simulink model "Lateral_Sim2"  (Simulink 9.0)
settings: Solver=ode45  StartTime=0.0  StopTime=80  RelTol=1e-3  EnableMultiTasking=on
InitFcn:
  | init_lat;
StopFcn:
  | pl
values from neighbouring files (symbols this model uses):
  Cyb = -0.023    [init_lat.m]    (also in init.m; init_pitch.m)
  Cyda = 0.0011    [init_lat.m]    (also in init.m; init_pitch.m)
  Cydr = 0.0034    [init_lat.m]    (also in init.m; init_pitch.m)
  d2r = pi/180    (= 0.0174532925199)    [frequ.m]    (also in init_lat.m; pl.m; init.m; freq.m)
  Mv = 1219.1    [init_lat.m]    (also in init.m; init_pitch.m)
  Qbar = 1220.6    [init_lat.m]    (also in init.m; init_pitch.m)
  Sref = 145.4    [init_lat.m]    (also in init.m; init_pitch.m)
undefined symbols (not defined in the file or in its folder): Al, Bl, Cl, Dl, Kpr

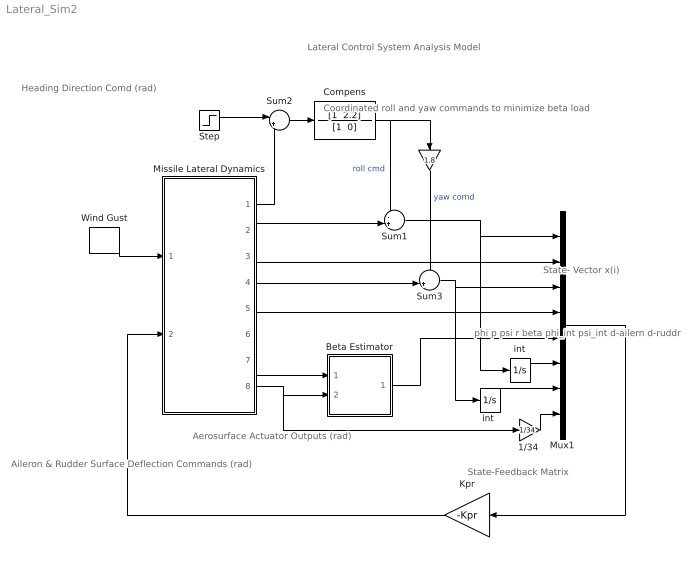
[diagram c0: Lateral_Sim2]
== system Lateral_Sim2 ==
  note: phi p psi r beta phi_int psi_int d-ailern d-ruddr
  note: Heading Direction Comd (rad)
  note: State- Vector x(i)
  note: Aileron & Rudder Surface Deflection Commands (rad)
  note: Aerosurface Actuator Outputs (rad)
  note: Coordinated roll and yaw commands to minimize beta load
  note: State-Feedback Matrix
  note: Lateral Control System Analysis Model
  " " : Gain  Gain=1.8
  "1/34 " : Gain  Gain=1/34
  Beta Estimator : Subsystem
  Compens : TransferFcn  Numerator="[1  2.2]"  Denominator="[1  0]"
  Kpr : Gain  Gain=-Kpr  Multiplication=Matrix(K*u)
  Missile Lateral Dynamics : Subsystem
  Mux1 : Mux  Inputs=[1, 1, 1, 1, 1, 1, 1, 2]
  Step : Step  Time=0  After=10*d2r  SampleTime=0
  Sum1 : Sum  Inputs=-+|
  Sum2 : Sum  Inputs=|+-
  Sum3 : Sum  Inputs=-+|
  Wind Gust : DiscretePulseGenerator  PulseType=Time based  Amplitude=30  Period=100  PulseWidth=5  PhaseDelay=10
  int : Integrator
  "int " : Integrator
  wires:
  Missile Lateral Dynamics/3(p) -> Mux1/2
  Missile Lateral Dynamics/5(r) -> Mux1/4
  Kpr/1 -> Missile Lateral Dynamics/2(aero)
  Sum1/1 -> Mux1/1, int/1
  Missile Lateral Dynamics/2(phi) -> Sum1/2
  Sum2/1 -> Compens/1
  int/1 -> Mux1/6
  Missile Lateral Dynamics/1(" Head") -> Sum2/2
  Compens/1 -> Sum1/1, " "/1  "roll cmd"
  Missile Lateral Dynamics/4(psi) -> Sum3/2
  Sum3/1 -> Mux1/3, "int "/1
  "int "/1 -> Mux1/7
  " "/1 -> Sum3/1  "yaw comd"
  Missile Lateral Dynamics/8(aeros) -> "1/34 "/1, Beta Estimator/2(delta)
  Mux1/1 -> Kpr/1
  "1/34 "/1 -> Mux1/8
  Missile Lateral Dynamics/7(Ny) -> Beta Estimator/1(Ny)
  Beta Estimator/1(beta) -> Mux1/5
  Wind Gust/1 -> Missile Lateral Dynamics/1(Gust)
  Step/1 -> Sum2/1

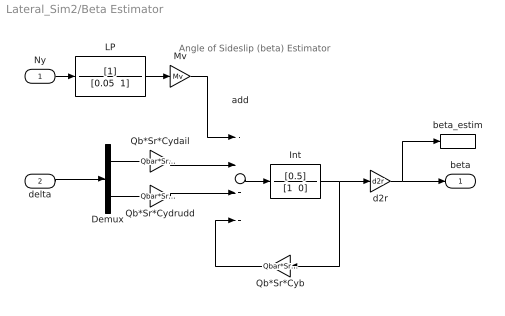
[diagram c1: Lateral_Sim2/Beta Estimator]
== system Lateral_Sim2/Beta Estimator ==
  note: Angle of Sideslip (beta) Estimator
  Ny : Inport
  delta : Inport  Port=2
  Demux : Demux  Outputs=2
  Int : TransferFcn  Numerator=[0.5]  Denominator="[1  0]"
  LP : TransferFcn  Denominator="[0.05  1]"
  Mv : Gain  Gain=Mv
  Qb*Sr*Cyb : Gain  Gain=Qbar*Sref*Cyb*1.2
  Qb*Sr*Cydail : Gain  Gain=Qbar*Sref*Cyda
  Qb*Sr*Cydrudd : Gain  Gain=Qbar*Sref*Cydr
  add : Sum  Inputs=-+++
  beta_estim : ToWorkspace  VariableName=betest  SampleTime=-1
  d2r : Gain  Gain=d2r
  beta : Outport
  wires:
  LP/1 -> Mv/1
  Qb*Sr*Cydail/1 -> add/2
  Qb*Sr*Cydrudd/1 -> add/3
  Qb*Sr*Cyb/1 -> add/4
  Ny/1 -> LP/1
  Int/1 -> d2r/1, Qb*Sr*Cyb/1
  d2r/1 -> beta_estim/1, beta/1
  Mv/1 -> add/1
  add/1 -> Int/1
  Demux/1 -> Qb*Sr*Cydail/1
  Demux/2 -> Qb*Sr*Cydrudd/1
  delta/1 -> Demux/1

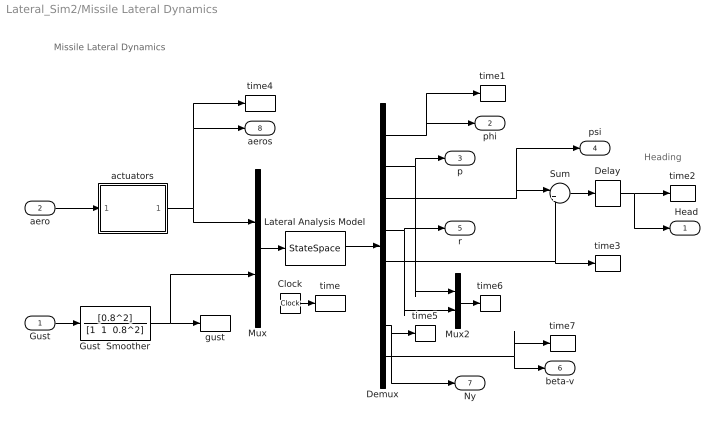
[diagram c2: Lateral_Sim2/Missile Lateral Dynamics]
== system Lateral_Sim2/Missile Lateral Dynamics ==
  note: Heading
  note: Missile Lateral Dynamics
  Gust : Inport
  aero : Inport  Port=2
  Clock : Clock
  Delay : TransportDelay  DelayTime=0.4  PadeOrder=2
  Demux : Demux  Outputs=8
  Gust  Smoother : TransferFcn  Numerator=[0.8^2]  Denominator="[1  1  0.8^2]"
  Lateral Analysis Model : StateSpace  A=Al  B=Bl  C=Cl  D=Dl  InitialCondition=0
  Mux : Mux  Inputs=[2, 1]
  Mux2 : Mux  Inputs=2
  Sum : Sum  Inputs=|++
  actuators : Subsystem
  gust : ToWorkspace  VariableName=gust  SampleTime=-1
  time : ToWorkspace  VariableName=time  SampleTime=-1
  time1 : ToWorkspace  VariableName=phi  SampleTime=-1
  time2 : ToWorkspace  VariableName=Head  SampleTime=-1
  time3 : ToWorkspace  VariableName=betai  SampleTime=-1
  time4 : ToWorkspace  VariableName=aeros  SampleTime=-1
  time5 : ToWorkspace  VariableName=Ay  SampleTime=-1
  time6 : ToWorkspace  VariableName=pr  SampleTime=-1
  time7 : ToWorkspace  VariableName=betav  SampleTime=-1
  " Head" : Outport
  phi : Outport  Port=2
  p : Outport  Port=3
  psi : Outport  Port=4
  r : Outport  Port=5
  beta-v : Outport  Port=6
  Ny : Outport  Port=7
  aeros : Outport  Port=8
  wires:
  Mux/1 -> Lateral Analysis Model/1
  Demux/1 -> time1/1, phi/1
  Demux/2 -> Mux2/1, p/1
  Demux/4 -> Mux2/2, r/1
  Demux/3 -> psi/1, Sum/1
  Demux/5 -> time3/1, Sum/2
  actuators/1("delo ") -> time4/1, aeros/1, Mux/1
  Sum/1 -> Delay/1
  aero/1 -> actuators/1(deli)
  Clock/1 -> time/1
  Gust/1 -> Gust  Smoother/1
  Demux/7 -> Ny/1, time5/1
  Mux2/1 -> time6/1
  Gust  Smoother/1 -> gust/1, Mux/2
  Lateral Analysis Model/1 -> Demux/1
  Demux/8 -> time7/1, beta-v/1
  Delay/1 -> " Head"/1, time2/1

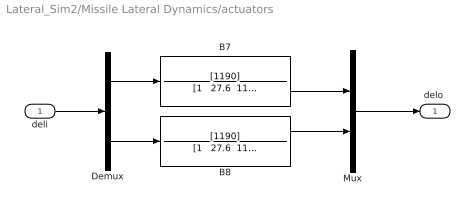
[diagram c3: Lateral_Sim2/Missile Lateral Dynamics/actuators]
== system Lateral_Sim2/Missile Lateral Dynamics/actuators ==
  deli : Inport
  B7 : TransferFcn  Numerator=[1190]  Denominator="[1   27.6  1190]"
  B8 : TransferFcn  Numerator=[1190]  Denominator="[1   27.6  1190]"
  Demux : Demux  Outputs=2
  Mux : Mux  Inputs=2
  "delo " : Outport
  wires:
  deli/1 -> Demux/1
  Demux/1 -> B7/1
  Demux/2 -> B8/1
  B8/1 -> Mux/2
  B7/1 -> Mux/1
  Mux/1 -> "delo "/1
